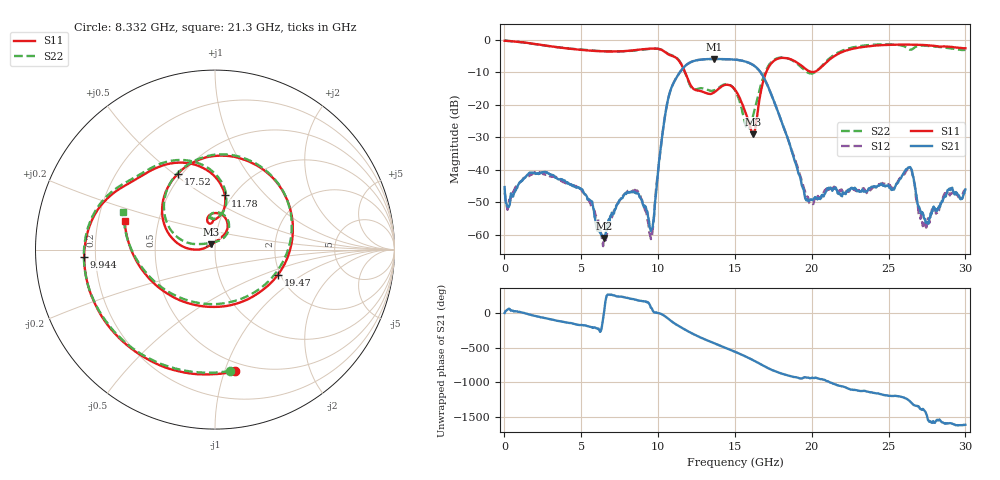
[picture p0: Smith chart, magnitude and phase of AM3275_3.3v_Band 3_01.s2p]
!Keysight Technologies,N5245B,MY58422270,A.16.20.02
!Date: Thursday, March 27, 2025 02:18:48
!Correction: S11(C  2-Port  )
!S21(C  2-Port  )
!S12(C  2-Port  )
!S22(C  2-Port  )
!S2P File: Measurements: S11, S21, S12, S22:
# Hz S  dB  R 50
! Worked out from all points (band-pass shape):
!   801 points, 10 MHz to 30 GHz, reference 50 ohm
!   highest |S21| = -5.88 dB at 13.66 GHz (marker M1); lowest = -61.0 dB at 6.458 GHz (marker M2)
!   |S21| within 3 dB of the highest: 11.59 GHz to 16.48 GHz (4.882 GHz wide, 34.8 % of centre)
!   lowest |S11| = -29.1 dB at 16.2 GHz (marker M3), VSWR 1.07, Z = 47.9 + j2.74 ohm
!   |S11| at or under -10 dB: 11.76 GHz to 17.03 GHz (5.274 GHz wide, 36.6 % of centre)
!   |S22| runs from -27.6 to -0.2 dB; largest |S21 - S12| = 0.0073
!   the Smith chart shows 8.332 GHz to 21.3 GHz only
!   S11 on the Smith chart (normalised r, x): 8.332 GHz: 0.43, -1.09; 9.944 GHz: 0.16, -0.03; 11.78 GHz: 0.92, +0.61; 17.52 GHz: 0.48, +0.52; 19.47 GHz: 1.95, -0.63; 21.3 GHz: 0.32, +0.14
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1e7  -0.29 -3.3  -45.32 -4.9  -47.02 -94.4  -0.19 -4.6
1.284575e9  -0.81 -82.7  -42.60 -6.2  -42.44 -3.3  -0.85 -83.2
2.671612e9  -1.77 -160.4  -40.64 -77.7  -41.51 -79.5  -1.79 -161.4
5.033325e9  -3.11 87.7  -45.94 -176.5  -46.50 -177.8  -3.04 86.2
6.45785e9  -3.57 20.0  -60.99 -38.7  -61.89 -146.8  -3.52 18.1
8.332225e9  -3.27 -80.5  -46.88 -165.1  -46.46 -167.3  -3.34 -82.9
9.531825e9  -2.70 -150.9  -58.84 69.2  -61.33 121.3  -2.73 -152.5
9.944188e9  -2.73 -176.6  -43.27 -4.2  -42.73 -4.8  -2.72 -178.1
1.001916e10  -2.79 178.5  -39.50 -6.5  -39.52 -7.0  -2.77 177.2
1.178108e10  -10.26 79.7  -7.95 112.7  -7.96 112.7  -10.41 77.9
1.275575e10  -15.75 93.4  -6.10 4.7  -6.10 4.7  -14.89 97.3
1.365545e10  -16.15 104.5  -5.88 -79.1  -5.88 -79.2  -15.53 99.7
1.5005e10  -15.34 67.1  -6.09 159.7  -6.09 159.8  -15.54 62.5
1.62046e10  -29.09 125.5  -7.81 36.8  -7.80 36.7  -22.99 153.5
1.751666e10  -6.55 116.1  -18.64 -110.7  -18.64 -111.1  -6.25 111.6
1.946601e10  -8.46 -21.7  -45.84 150.6  -45.23 136.1  -9.08 -27.6
2.002832e10  -9.91 -82.4  -49.33 149.5  -50.29 147.5  -10.33 -92.2
2.13029e10  -5.55 162.4  -46.09 72.2  -45.90 67.9  -5.16 157.5
2.501416e10  -1.56 38.1  -44.78 -109.5  -44.60 -106.2  -1.40 34.8
2.64012e10  -1.48 4.4  -39.14 168.4  -39.16 169.4  -3.03 2.5
2.737588e10  -1.62 -21.5  -55.14 27.4  -57.20 -97.7  -1.80 -21.2
3e10  -2.60 -113.3  -46.05 -166.3  -46.09 -166.8  -3.11 -115.0
